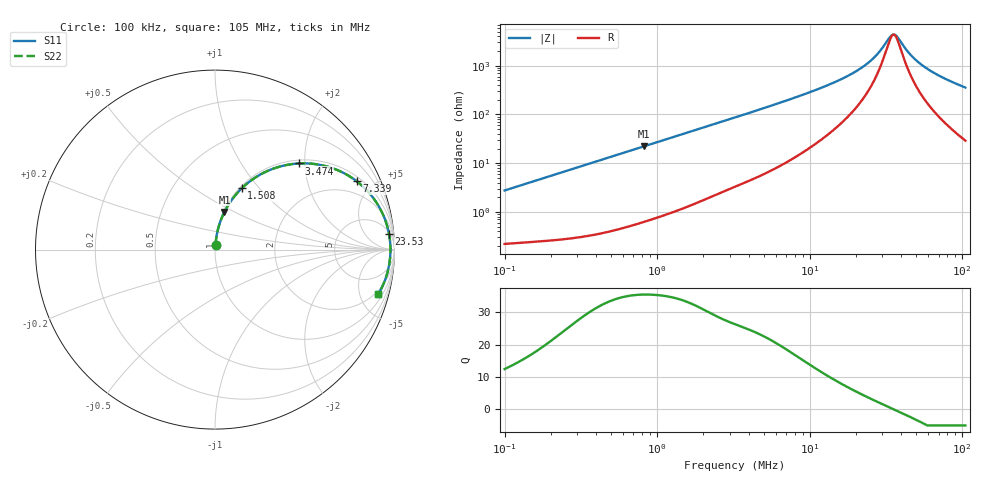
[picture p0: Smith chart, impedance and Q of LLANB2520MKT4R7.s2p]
! LLANB2520MKT4R7  S-PARAMETER MODEL  ( General Type )
! Model Generated by TAIYO YUDEN Corporation (http://www.ty-top.com)
! Version 2.0
! TAIYO YUDEN Control No. 20210629
! Copyright(c) 2012 TAIYO YUDEN CO.,LTD. All Rights Reserved.
! Product Description (link to TY-COMPAS)
! https://ds.yuden.co.jp/TYCOMPAS/or/detail?pn=LLANB2520MKT4R7M&u=M
! Products Name : Inductors
! Characteristics :
!  Inductance : 4.7 uH , SRF(min) : -Hz , DC Resistance(max) : 0.26 Ohm
!  Rated Current : Saturation :1500 mA , Temp Rise : 1300 mA (40 degC)
!  Case Size : 2.5 x 2.0 / 0.098 x 0.079 [mm/inch] , Thickness : 1.2 / 0.047 [mm/inch]
!  (Conditions: Temperature = 25 degC , DC Bias Current/Voltage = 0A / 0V)
! External Node Assignments :
!  1  o---GGG---o  2
! GND o---------o GND
! Frequency Range : 0.1MHz  -  105.0131MHz  [ 402 STEP ]
# MHz S RI R 50
! Freq[MHz].  S11 Real  S11 Imag  S21 Real  S21 Imag  S12 Real  S12 Imag  S22 Real  S22 Imag
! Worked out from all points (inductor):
!   401 points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, 100 kHz to 105 MHz, reference 50 ohm
!   read as one part in series: L = 4.36 uH near 103.5 kHz
!   highest Q = 35.6 at 820.2 kHz (marker M1), where L = 4.3 uH
!   self-resonance near 35.55 MHz
!   S11 on the Smith chart (normalised r, x): 100 kHz: 1.00, +0.05; 1.508 MHz: 1.02, +0.81; 3.474 MHz: 1.07, +1.86; 7.339 MHz: 1.22, +4.03; 23.53 MHz: 6, +21; 105 MHz: 1.58, -7.11
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0.1  0.00295 0.0273  0.9971 -0.0273  0.9971 -0.0273  0.00295 0.0273
0.32067  0.0106 0.0861  0.9894 -0.0861  0.9894 -0.0861  0.0106 0.0861
0.820212  0.0523 0.2089  0.9477 -0.2089  0.9477 -0.2089  0.0523 0.2089
1.028292  0.0777 0.2539  0.9223 -0.2539  0.9223 -0.2539  0.0777 0.2539
1.507596  0.1486 0.3411  0.8514 -0.3411  0.8514 -0.3411  0.1486 0.3411
2.172202  0.2605 0.4226  0.7395 -0.4226  0.7395 -0.4226  0.2605 0.4226
3.297424  0.4403 0.4777  0.5597 -0.4777  0.5597 -0.4777  0.4403 0.4777
3.474035  0.4653 0.4798  0.5347 -0.4798  0.5347 -0.4798  0.4653 0.4798
4.919221  0.6313 0.461  0.3687 -0.461  0.3687 -0.461  0.6313 0.461
7.338678  0.79 0.3805  0.21 -0.3805  0.21 -0.3805  0.79 0.3805
10.39154  0.8819 0.2875  0.1181 -0.2875  0.1181 -0.2875  0.8819 0.2875
16.91091  0.9496 0.1613  0.0504 -0.1613  0.0504 -0.1613  0.9496 0.1613
23.53294  0.9698 0.086  0.0302 -0.086  0.0302 -0.086  0.9698 0.086
28.00317  0.9751 0.0491  0.0249 -0.0491  0.0249 -0.0491  0.9751 0.0491
33.32256  0.9775 0.0133  0.0225 -0.0133  0.0225 -0.0133  0.9775 0.0133
35.10732  0.9777 0.00259  0.0223 -0.00259  0.0223 -0.00259  0.9777 0.00259
36.98767  0.9777 -0.00807  0.0223 0.00807  0.0223 0.00807  0.9777 -0.00807
47.18462  0.9743 -0.0584  0.0257 0.0584  0.0257 0.0584  0.9743 -0.0584
52.37441  0.9711 -0.0806  0.0289 0.0806  0.0289 0.0806  0.9711 -0.0806
60.19272  0.965 -0.1111  0.035 0.1111  0.035 0.1111  0.965 -0.1111
78.1341  0.9464 -0.1723  0.0536 0.1723  0.0536 0.1723  0.9464 -0.1723
105.0131  0.9098 -0.2486  0.0902 0.2486  0.0902 0.2486  0.9098 -0.2486
